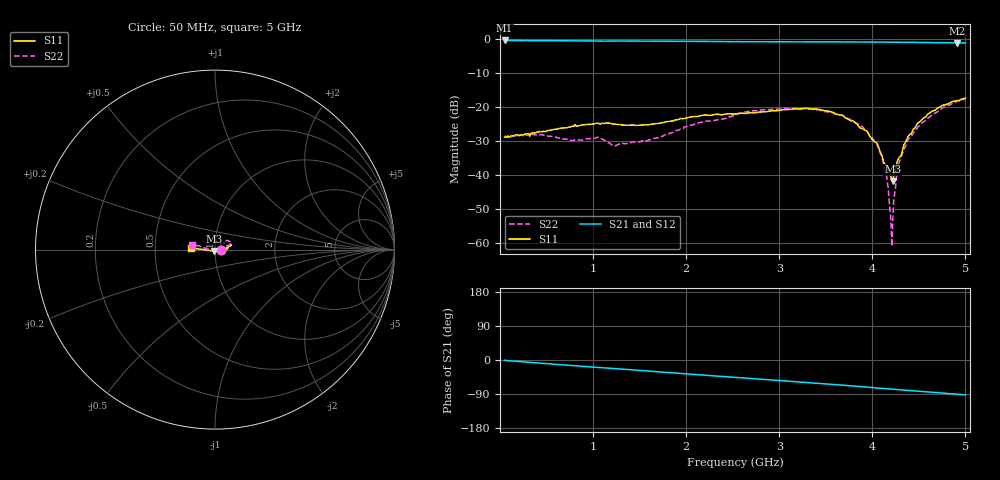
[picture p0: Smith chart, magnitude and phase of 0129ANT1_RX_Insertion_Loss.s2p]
! MASWSS0129 de-embedded Sparameters using port extention method. ANT1 to RX Insertion Loss using 3 volt control
! Board loss is removed and phase length of connector and line length of board are dialed out
! 100pF blocking capacitor
! Sample board 1000013136
#	Hz	S	DB	R	50
!	Freq	S11	S21	S12	S22
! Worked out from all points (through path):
!   401 points, 50 MHz to 5 GHz, reference 50 ohm
!   highest |S21| = -0.52 dB at 50 MHz (marker M1); lowest = -1.3 dB at 4.91 GHz (marker M2)
!   group delay of S21, straight-line fit = 50.5 ps
!   lowest |S11| = -42.0 dB at 4.22 GHz (marker M3), VSWR 1.02, Z = 49.7 - j0.738 ohm
!   |S11| at or under -10 dB: start of sweep to end of sweep
!   |S22| runs from -61.1 to -17.7 dB; largest |S21 - S12| = 0.01
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5e7  -28.96 -2.8  -0.52 -0.8  -0.45 -1.2  -28.83 -1.1
4.46e8  -27.34 4.1  -0.57 -8.6  -0.58 -8.6  -28.24 7.5
8.79e8  -25.41 -4.4  -0.66 -16.6  -0.64 -16.6  -29.84 15.6
1.05e9  -24.88 -2.8  -0.69 -19.7  -0.69 -19.7  -29.01 14.5
1.24e9  -25.17 -5.6  -0.69 -22.6  -0.71 -22.7  -31.52 17.8
1.7e9  -24.98 0.1  -0.74 -31.0  -0.74 -31.1  -29.13 41.3
2.53e9  -22.17 14.7  -0.88 -45.8  -0.88 -45.9  -22.52 39.4
3.35e9  -20.69 17.7  -0.93 -60.6  -0.95 -60.7  -20.81 19.1
3.68e9  -22.55 11.2  -0.96 -66.5  -0.96 -66.6  -22.55 17.9
3.99e9  -29.27 -9.0  -1.01 -72.3  -0.98 -72.5  -28.70 15.4
4.1e9  -34.16 -23.1  -1.00 -74.6  -1.00 -74.6  -34.52 10.4
4.15e9  -37.32 -50.7  -1.02 -75.6  -1.02 -75.6  -39.58 16.2
4.17e9  -38.42 -59.0  -1.02 -76.2  -1.01 -76.2  -43.71 11.4
4.18e9  -39.23 -65.0  -1.00 -76.3  -1.02 -76.5  -47.45 4.6
4.21e9  -41.45 -92.2  -1.03 -76.7  -1.01 -76.9  -61.06 -106.0
4.22e9  -41.96 -111.4  -1.03 -77.2  -1.02 -77.2  -53.32 -156.6
4.27e9  -35.94 -148.0  -1.05 -78.1  -1.05 -78.1  -38.78 179.5
4.29e9  -34.94 -155.9  -1.05 -78.5  -1.05 -78.7  -36.20 -177.2
4.39e9  -28.50 -173.2  -1.06 -80.5  -1.07 -80.6  -29.37 176.5
4.6e9  -22.11 178.8  -1.14 -84.5  -1.12 -84.6  -23.33 168.8
4.91e9  -18.24 176.4  -1.26 -90.3  -1.23 -90.5  -18.47 167.5
5e9  -17.49 175.7  -1.26 -92.1  -1.27 -92.3  -17.70 167.4
